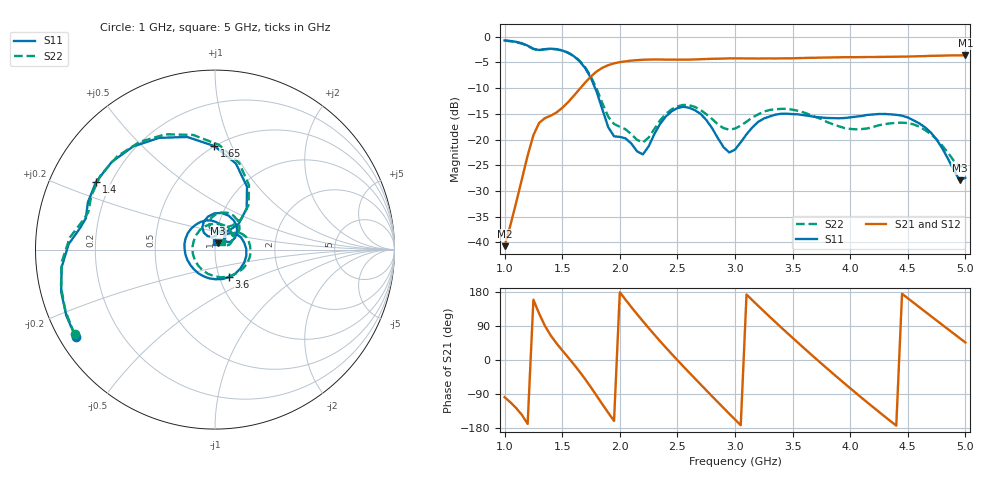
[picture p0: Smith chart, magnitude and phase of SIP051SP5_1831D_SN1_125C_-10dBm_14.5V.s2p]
# GHz  S  dB  R  50
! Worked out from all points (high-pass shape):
!   81 points, 1 GHz to 5 GHz, reference 50 ohm
!   highest |S21| = -3.63 dB at 5 GHz (marker M1); lowest = -40.7 dB at 1 GHz (marker M2)
!   |S21| within 3 dB of the highest: 1.809 GHz to end of sweep
!   lowest |S11| = -27.9 dB at 4.95 GHz (marker M3), VSWR 1.08, Z = 51.7 + j3.7 ohm
!   |S11| at or under -10 dB: 1.785 GHz to end of sweep
!   |S22| runs from -25.2 to -0.8 dB; largest |S21 - S12| = 0.0016
!   S11 on the Smith chart (normalised r, x): 1 GHz: 0.05, -0.29; 1.4 GHz: 0.14, +0.26; 1.65 GHz: 0.50, +0.86; 3.6 GHz: 1.11, -0.35; 5 GHz: 1.01, +0.09
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1  -0.75 -147.7  -40.73 -98.2  -40.84 -98.6  -0.78 -148.9
1.25  -2.37 170.9  -19.16 159.0  -19.13 158.8  -2.41 168.2
1.4  -2.36 150.4  -15.37 64.9  -15.36 65.1  -2.38 147.2
1.65  -4.78 90.3  -10.21 -30.4  -10.20 -30.3  -4.67 87.7
1.7  -6.13 76.4  -8.92 -50.7  -8.92 -50.8  -5.99 74.5
1.85  -14.26 47.4  -6.05 -117.3  -6.03 -117.3  -13.02 49.3
2  -19.49 77.2  -4.97 178.8  -4.96 178.7  -17.53 67.6
2.2  -22.89 103.5  -4.51 102.6  -4.51 102.6  -20.58 87.5
2.35  -16.95 119.8  -4.45 49.6  -4.44 49.6  -16.27 102.0
2.55  -13.64 79.5  -4.48 -16.5  -4.47 -16.4  -13.28 71.0
2.75  -16.18 37.6  -4.36 -79.7  -4.36 -79.7  -15.06 39.7
3  -21.97 50.3  -4.24 -157.1  -4.23 -157.1  -17.89 40.9
3.15  -17.67 45.0  -4.25 157.9  -4.25 157.9  -15.73 35.4
3.3  -15.54 13.4  -4.24 114.4  -4.25 114.4  -14.26 15.0
3.6  -15.29 -62.8  -4.16 31.1  -4.17 31.0  -14.78 -42.6
3.7  -15.63 -88.2  -4.12 4.0  -4.11 4.1  -15.63 -66.3
4.05  -15.56 -169.1  -4.00 -87.2  -3.99 -87.2  -18.02 -169.9
4.35  -15.11 127.9  -3.93 -161.3  -3.94 -161.2  -16.86 102.1
4.5  -15.72 97.5  -3.88 162.9  -3.87 163.0  -16.81 66.9
4.7  -18.65 60.3  -3.74 116.0  -3.74 116.0  -18.96 30.7
4.95  -27.93 62.9  -3.65 57.8  -3.65 57.9  -25.23 34.4
5  -27.44 84.1  -3.63 46.3  -3.64 46.2  -25.02 46.2
